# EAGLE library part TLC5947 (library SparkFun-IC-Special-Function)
TI TLC5947 24-channel 12-bit constant current PWM driver The TLC5947 is a 24-channel, constant-current sink LED driver. Each channel is individually adjustable with 4096 pulse-width modulated (PWM) steps. PWM control is repeated automatically with the programmed grayscale (GS) data. GS data are written via a serial interface port. The current value of all 24 channels is set by a single external resistor. The TLC5947 has a thermal shutdown (TSD) function that turns off all output drivers during an over-temperature condition. All of the output drivers automatically restart when the temperature returns to normal conditions. SparkFun Products: [PRODUCT 1]
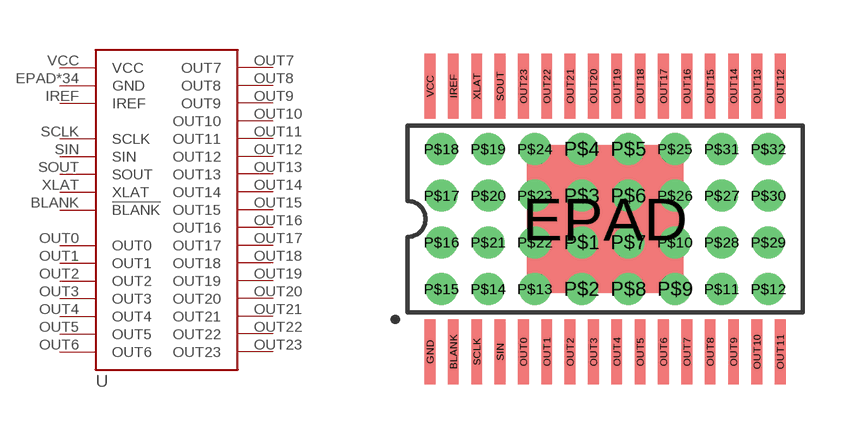
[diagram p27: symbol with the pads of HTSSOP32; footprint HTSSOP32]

Designator prefix -

## TLC5947 (PROD_ID: IC-13817)  [HTSSOP32]
BLANK  !BLANK
EPAD  GND  pwr
GND  GND  pwr
IREF  IREF
OUT0  OUT0  out
OUT1  OUT1  out
OUT2  OUT2  out
OUT3  OUT3  out
OUT4  OUT4  out
OUT5  OUT5  out
OUT6  OUT6  out
OUT7  OUT7  out
OUT8  OUT8  out
OUT9  OUT9  out
OUT10  OUT10  out
OUT11  OUT11  out
OUT12  OUT12  out
OUT13  OUT13  out
OUT14  OUT14  out
OUT15  OUT15  out
OUT16  OUT16  out
OUT17  OUT17  out
OUT18  OUT18  out
OUT19  OUT19  out
OUT20  OUT20  out
OUT21  OUT21  out
OUT22  OUT22  out
OUT23  OUT23  out
P$1  GND  pwr
P$2  GND  pwr
P$3  GND  pwr
P$4  GND  pwr
P$5  GND  pwr
P$6  GND  pwr
P$7  GND  pwr
P$8  GND  pwr
P$9  GND  pwr
P$10  GND  pwr
P$11  GND  pwr
P$12  GND  pwr
P$13  GND  pwr
P$14  GND  pwr
P$15  GND  pwr
P$16  GND  pwr
P$17  GND  pwr
P$18  GND  pwr
P$19  GND  pwr
P$20  GND  pwr
P$21  GND  pwr
P$22  GND  pwr
P$23  GND  pwr
P$24  GND  pwr
P$25  GND  pwr
P$26  GND  pwr
P$27  GND  pwr
P$28  GND  pwr
P$29  GND  pwr
P$30  GND  pwr
P$31  GND  pwr
P$32  GND  pwr
SCLK  SCLK
SIN  SIN
SOUT  SOUT
VCC  VCC  pwr
XLAT  XLAT

## Footprint HTSSOP32 (pad centres in mm)
[HTSSOP-32] - [Package for the TLC5947 PWM driver] Specifications: Pin count: [32] Pin pitch: [0.65 mm] Area: [11.00 mm x 6.20 mm] Datasheet referenced for footprint Example device(s): [TLC5947]
smd 0.3 x 1.8: BLANK -4.225,-3.7; GND -4.875,-3.7; IREF -4.225,3.7; OUT0 -2.275,-3.7; OUT1 -1.625,-3.7; OUT2 -0.975,-3.7; OUT3 -0.325,-3.7; OUT4 0.325,-3.7; OUT5 0.975,-3.7; OUT6 1.625,-3.7; OUT7 2.275,-3.7; OUT8 2.925,-3.7; OUT9 3.575,-3.7; OUT10 4.225,-3.7; OUT11 4.875,-3.7; OUT12 4.875,3.7; OUT13 4.225,3.7; OUT14 3.575,3.7; OUT15 2.925,3.7; OUT16 2.275,3.7; OUT17 1.625,3.7; OUT18 0.975,3.7; OUT19 0.325,3.7; OUT20 -0.325,3.7; OUT21 -0.975,3.7; OUT22 -1.625,3.7; OUT23 -2.275,3.7; SCLK -3.575,-3.7; SIN -2.925,-3.7; SOUT -2.925,3.7; VCC -4.875,3.7; XLAT -3.575,3.7
smd 4.36 x 4.11: EPAD 0,0
drill 0.381: P$1 -0.65,-0.65; P$2 -0.65,-1.95; P$3 -0.65,0.65; P$4 -0.65,1.95; P$5 0.65,1.95; P$6 0.65,0.65; P$7 0.65,-0.65; P$8 0.65,-1.95; P$9 1.95,-1.95; P$10 1.95,-0.65; P$11 3.25,-1.95; P$12 4.55,-1.95; P$13 -1.95,-1.95; P$14 -3.25,-1.95; P$15 -4.55,-1.95; P$16 -4.55,-0.65; P$17 -4.55,0.65; P$18 -4.55,1.95; P$19 -3.25,1.95; P$20 -3.25,0.65; P$21 -3.25,-0.65; P$22 -1.95,-0.65; P$23 -1.95,0.65; P$24 -1.95,1.95; P$25 1.95,1.95; P$26 1.95,0.65; P$27 3.25,0.65; P$28 3.25,-0.65; P$29 4.55,-0.65; P$30 4.55,0.65; P$31 3.25,1.95; P$32 4.55,1.95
